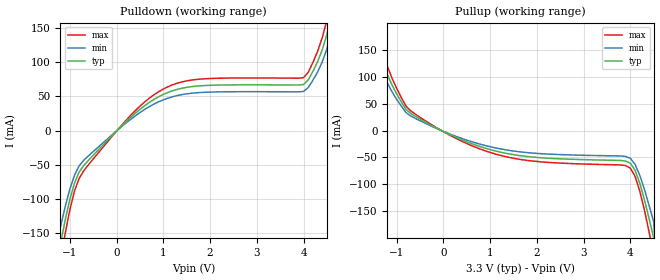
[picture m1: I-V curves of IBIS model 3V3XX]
[IBIS Ver]   2.1
[File name]   ics571_3.ibs
[File Rev]   2.0
[Date]   9/13/2000
[Source]   ICS MicroClock Applications Engineering 2
[Disclaimer] This information is for modeling purposes only, and is
(C) Copyright Integrated Circuit Systems, Inc. 1997-2001
   All rights reserved
ICS hereby grants the user of this IBIS model a non-exclusive,
nontransferable license to use this IBIS model under the following terms.
Before using this IBIS model, the user should read this license.
If the user does not accept these terms,  the IBIS model should be
returned to ICS within 30 days.
   The user is granted this license only to use the IBIS model and
is not granted rights to sell, load, rent, lease or license the IBIS
model in whole or in part, or in modified form to anyone other than
user. User may modify the IBIS model to suit its specific
applications but rights to derivative works and such modifications
shall belong to ICS.
   This IBIS model is provided on an "AS IS" basis and ICS makes
absolutely no warranty with respect to the information contained
herein. ICS DISCLAIMS AND CUSTOMER WAIVES ALL WARRANTIES, EXPRESS
OR IMPLIED, INCLUDING WARRANTIES OF MERCHANTABILITY OR FITNESS FOR
A PARTICULAR PURPOSE. The entire risk as to quality and performance
is with the Customer. ACCORDINGLY, IN NO EVENT SHALL THE COMPANY BE
LIABLE FOR ANY DAMAGES, WHETHER IN CONTRACT OR TORT,INCLUDING ANY
LOST PROFITS OR OTHER INCIDENTAL, CONSEQUENTIAL, EXEMPLARY, OR
PUNITIVE DAMAGES ARISING OUT OF THE USE OR APPLICATION OF THE IBIS
model provided in this package. Further, ICS reserves the right to
make changes without notice to any product herein to improve
reliability, function, or design. ICS does not convey any license
under patent rights or any other intellectual property rights,
including those of third parties.
   ICS is not obligated to provide maintenance or support
for the licensed IBIS model.
[Component]   ics571
[Manufacturer] Integrated Circuit Systems Inc.
[Package]
|   typ   min   max
R_pkg   40m   35m   45m
L_pkg   1.65nH   1.35nH   1.95nH
C_pkg   0.24pF   0.14pF   0.34pF
[pin]   signal_name   model_name   R_pin   L_pin   C_pin
   7   CLK   3V3XX
   4   CLK/2   3V3XX
| Models and submodels in the file (1): 3V3XX (Output)
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|   ICS571 3V Clock Drive Model
| This model is suitable for all output pins on the
| ICS571
[Model]   3V3XX
Model_type   Output
Polarity   Non-Inverting
|   typ   min   max
C_comp   5pF   4pF   6pF
|   typ   min   max
[Voltage range]  3.3V   3.15V   3.45V
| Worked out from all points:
|   slope of the pulldown table from 0 to 0.495 V, typ, clamps not added: 15.7 ohm
|   slope of the pullup table from 0 to 0.495 V, typ, clamps not added: 26.1 ohm
[pulldown]
|Voltage I (typ)   I (min)   I (max)
-3.3V     -3A        -3A        -3A
-1.3V     -199.9mA   -169.9mA   -229.9mA
-1.1V     -132mA     -112.2mA   -151.8mA
-900mV    -77.23mA   -65.65mA   -88.82mA
-700mV    -51.19mA   -43.51mA   -58.87mA
400mV     25.31mA    21.51mA    29.1mA
1.1V      55.9mA     47.52mA    64.28mA
4V        67.53mA    57.4mA     77.66mA
4.5V      140.8mA    119.7mA    161.9mA
4.6V      173.4mA    147.4mA    199.5mA
4.7V      200.4mA    170.3mA    230.4mA
6.6V      3A         3A         3A
[pullup]
|Voltage I (typ)   I (min)   I (max)
-3.3V     3A         3A         3A
-1.5V     200.3mA    170.3mA    230.4mA
-1.4V     161.7mA    137.4mA    185.9mA
-1.2V     103.9mA    88.33mA    119.5mA
-800mV    39.29mA    33.4mA     45.19mA
200mV     -10.06mA   -8.55mA    -11.57mA
1.6V      -46.18mA   -39.25mA   -53.1mA
4V        -60.82mA   -51.69mA   -69.94mA
4.2V      -97.59mA   -82.95mA   -112.2mA
4.4V      -163.8mA   -139.2mA   -188.4mA
4.5V      -199.9mA   -169.9mA   -229.9mA
6.6V      -3A        -3A        -3A
[Ramp]
|   typ   min   max
dV/dt_r   2.5/0.7n   2.2/0.7n   2.7/0.7n
dV/dt_f   2.5/0.6n   2.2/0.6n   2.7/0.6n
